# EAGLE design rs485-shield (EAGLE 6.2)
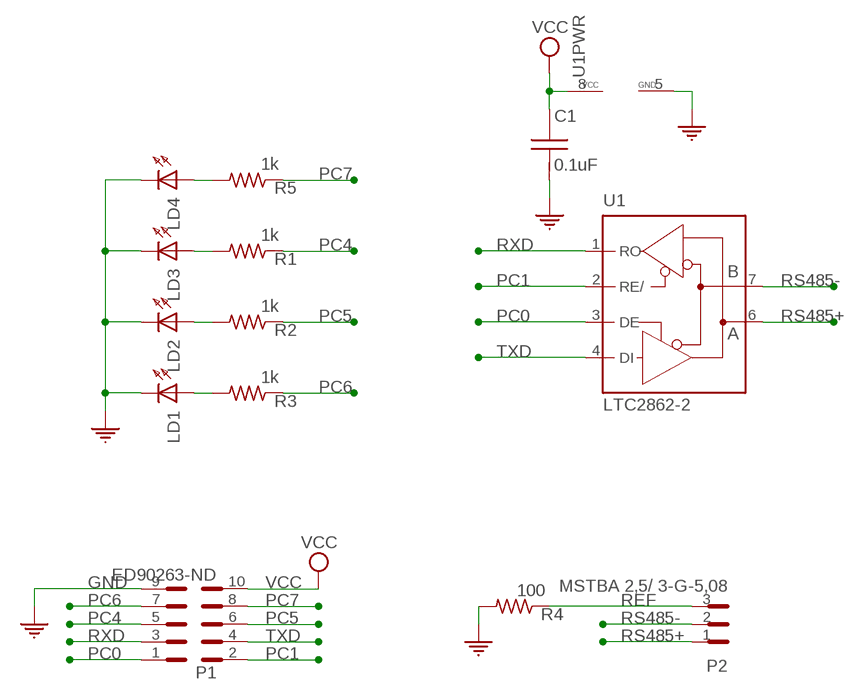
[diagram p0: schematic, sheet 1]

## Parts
C1  0.1uF  C-US-0805  [C0805]
LD1  LED-3MM  [LED-3MM]
LD2  LED-3MM  [LED-3MM]
LD3  LED-3MM  [LED-3MM]
LD4  LED-3MM  [LED-3MM]
P1  ED90263-ND  PINHEADER2X5-0.1"SPACING  [PINHD2X5]
P2  MSTBA 2,5/ 3-G-5,08  PINHEADER1X3-MSTBA  [CON-MSTBA]
R1  1k  R_-RES50/500_  [RES50/500]
R2  1k  R_-RES50/500_  [RES50/500]
R3  1k  R_-RES50/500_  [RES50/500]
R4  100  R_-RES50/500_  [RES50/500]
R5  1k  R_-RES50/500_  [RES50/500]
U1  LTC2862-2  RS485-TRANSCEIVER-SOP8  [SOP08]

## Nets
GND: C1.2 LD1.C LD2.C LD3.C LD4.C P1.9 R4.2 U1.5(GND)
N$2: LD4.A R5.2
N$8: LD3.A R1.2
N$9: LD2.A R2.2
N$10: LD1.A R3.2
PC0: P1.1 U1.3(DE)
PC1: P1.2 U1.2(RE/)
PC4: P1.5 R1.1
PC5: P1.6 R2.1
PC6: P1.7 R3.1
PC7: P1.8 R5.1
REF: P2.3 R4.1
RS485+: P2.1 U1.6(A)
RS485-: P2.2 U1.7(B)
RXD: P1.3 U1.1(RO)
TXD: P1.4 U1.4(DI)
VCC: C1.1 P1.10 U1.8(VCC)

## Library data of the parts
C1 = TWS:C-US: Cap non pol.
LD1-LD4 = TWS:LED: Single LED
P1 = TWS:PINHEADER2X5: Pinheader 2x5 Last modified 08-19-2004: Added Footprint 0.1" Spacing 07-29-2004: Added Foot Print for AVR-JTAG
P2 = TWS:PINHEADER1X3: Last edited 09-25-2004: Added Package CON-703W-00/54
R1-R5 = TWS:R_?_*
U1 = TWS:RS485-TRANSCEIVER: RS485 Transceiver/Driver MAX481/75XX184/Etc. Created 08-16-2004

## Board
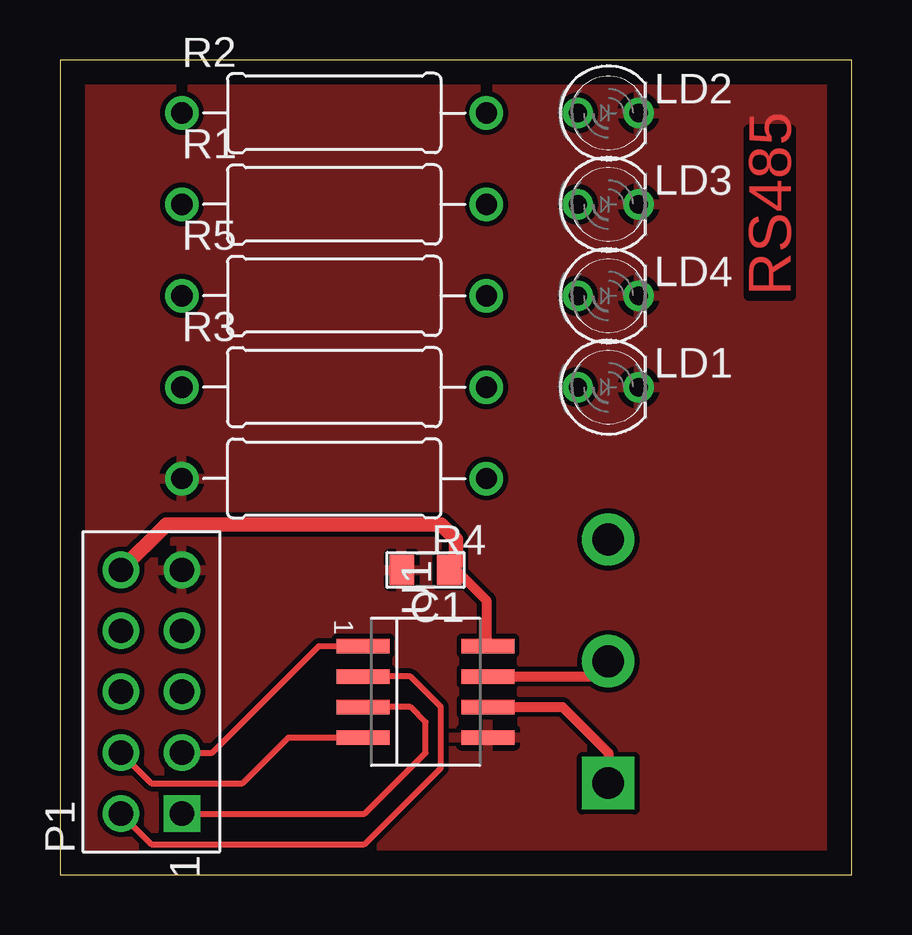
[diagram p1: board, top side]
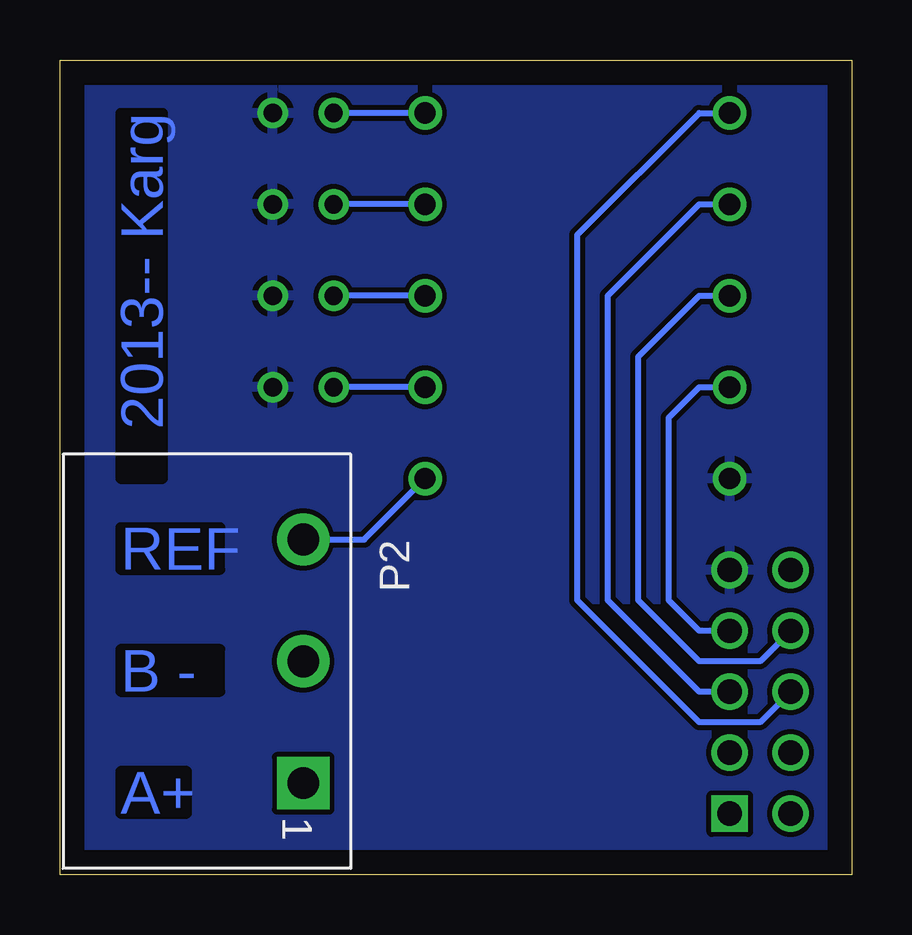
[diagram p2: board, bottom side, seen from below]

Size 33 x 33.96 mm. Coordinates in mm from the lower left corner, seen from the top.
Outline: 0,0 33,0 33,33.96 0,33.96 0,0
Copper layers (1*16): Top_Copper 0.035mm / dielectric 1.5mm / Bottom_Copper 0.035mm
Design rules: minimum track width 10mil, minimum drill 0.6mm, track to track 8mil, track to pad 8mil, pad to pad 8mil, via to via 8mil, smd to smd 8mil, copper to edge 40mil, drill to drill 8mil, minimum pad ring 10mil, minimum via ring 8mil, stop-mask expansion 4mil, vias tented up to drill 0mil, thermal gap 10mil

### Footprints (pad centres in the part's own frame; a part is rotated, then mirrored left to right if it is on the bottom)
C0805 = smd 1.016 x 1.27: 1 -0.991,0; 2 0.991,0
LED-3MM = drill 0.762: A -1.27,0; C 1.27,0
PINHD2X5 = drill 1.016 square: 1 -5.08,-1.27 | drill 1.016: 2 -5.08,1.27; 3 -2.54,-1.27; 4 -2.54,1.27; 5 0,-1.27; 6 0,1.27; 7 2.54,-1.27; 8 2.54,1.27; 9 5.08,-1.27; 10 5.08,1.27
CON-MSTBA = drill 1.321 pad 2.184 square: 1 5.08,0 | drill 1.321 pad 2.184: 2 0,0; 3 -5.08,0
RES50/500 = drill 0.889: 1 -6.35,0; 2 6.35,0
SOP08 = smd 0.6 x 2.2: 1 -1.905,-2.6; 2 -0.635,-2.6; 3 0.635,-2.6; 4 1.905,-2.6; 5 1.905,2.6; 6 0.635,2.6; 7 -0.635,2.6; 8 -1.905,2.6

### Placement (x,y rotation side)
C1  15.24,12.7 180 top
LD1  22.86,20.32 0 top
LD2  22.86,31.75 0 top
LD3  22.86,27.94 0 top
LD4  22.86,24.13 0 top
P1  3.81,7.62 90 top
P2  22.86,8.89 270 bottom
R1  11.43,27.94 0 top
R2  11.43,31.75 0 top
R3  11.43,20.32 0 top
R4  11.43,16.51 180 top
R5  11.43,24.13 0 top
U1  15.24,7.62 270 top

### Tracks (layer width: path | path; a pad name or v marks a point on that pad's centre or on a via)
GND
  pour Bottom_Copper: 0,34.29 33.02,34.29 33.02,0 0,0
  pour Top_Copper: 0,34.29 33.02,34.29 33.02,0 0,0
N$2
  Bottom_Copper 0.254: R5.2 LD4.A
N$8
  Bottom_Copper 0.254: R1.2 LD3.A
N$9
  Bottom_Copper 0.254: R2.2 LD2.A
N$10
  Bottom_Copper 0.254: R3.2 LD1.A
PC0
  Top_Copper 0.254: P1.1 12.7,2.54 15.24,5.08 15.24,6.35 14.61,6.99 U1.3
PC1
  Top_Copper 0.254: P1.2 3.81,1.27 12.7,1.27 15.88,4.45 15.88,6.99 14.61,8.26 U1.2
PC4
  Bottom_Copper 0.254: P1.5 6.35,7.62 10.16,11.43 10.16,24.13 6.35,27.94 R1.1
PC5
  Bottom_Copper 0.254: P1.6 3.81,6.35 6.35,6.35 11.43,11.43 11.43,26.67 6.35,31.75 R2.1
PC6
  Bottom_Copper 0.254: R3.1 6.35,20.32 7.62,19.05 7.62,11.43 6.35,10.16 P1.7
PC7
  Bottom_Copper 0.254: R5.1 6.35,24.13 8.89,21.59 8.89,11.43 6.35,8.89 3.81,8.89 P1.8
REF
  Bottom_Copper 0.254: R4.1 20.32,13.97 P2.3
RS485+
  Top_Copper 0.406: U1.6 20.95,6.99 22.86,5.08 P2.1
RS485-
  Top_Copper 0.406: U1.7 22.23,8.26 P2.2
RXD
  Top_Copper 0.254: P1.3 6.35,5.08 10.79,9.53 U1.1
TXD
  Top_Copper 0.254: P1.4 3.81,3.81 7.62,3.81 9.53,5.71 U1.4
VCC
  Top_Copper 0.406: C1.1 16.51,12.7 17.78,11.43 17.78,9.59 U1.8
  Top_Copper 0.61: P1.10 4.45,14.61 15.88,14.61 16.51,13.97 16.51,12.98 C1.1

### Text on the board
Top_Copper: RS485
Bottom_Copper: 2013-- Karg | REF | B - | A+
